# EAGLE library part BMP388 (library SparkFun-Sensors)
Bosch BMP3388 Pressure Sensor Senses pressure from 300 hPa to 1250 hPa, sends data out over I2C or Serial
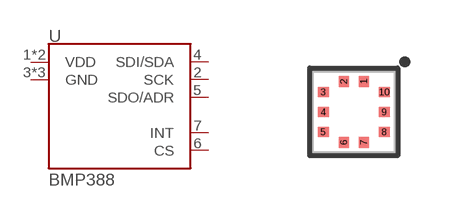
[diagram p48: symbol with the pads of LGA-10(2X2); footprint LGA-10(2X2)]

Designator prefix U

## BMP388BMP388 (PROD_ID: IC-14045)  [LGA-10(2X2)]
1  VDD
2  SCK
3  GND
4  SDI/SDA
5  SDO/ADR
6  CS
7  INT
8  GND
9  GND
10  VDD

## Footprint LGA-10(2X2) (pad centres in mm)
LGA10 Specifications: Pin count: 10 Pin pitch: .5mm Area: 2.0 x 2.0 mm Datasheet referenced for footprint
smd 0.25 x 0.275: 1 0.25,0.762; 2 -0.25,0.762; 6 -0.25,-0.762; 7 0.25,-0.762
smd 0.275 x 0.25: 3 -0.762,0.5; 4 -0.762,0; 5 -0.762,-0.5; 8 0.762,-0.5; 9 0.762,0; 10 0.762,0.5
